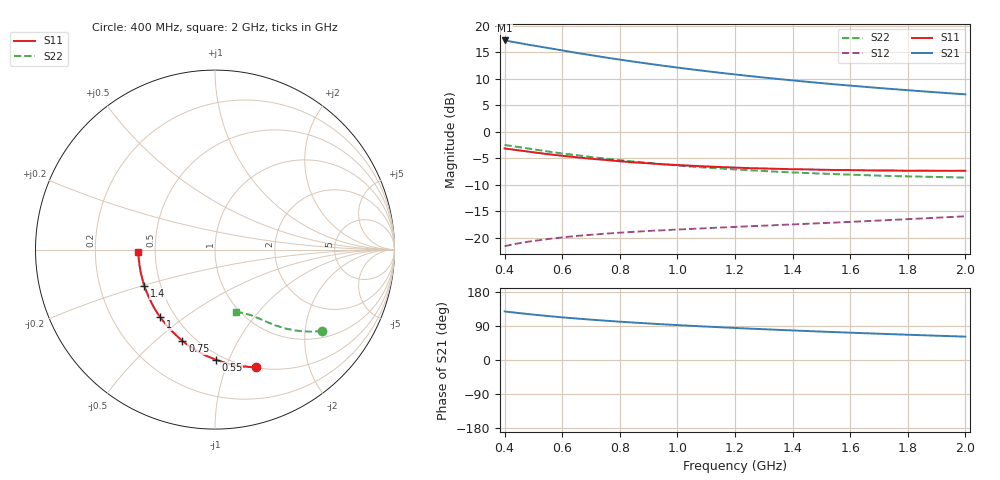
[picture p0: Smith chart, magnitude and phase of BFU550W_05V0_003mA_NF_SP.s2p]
! Filename:  P:\Prog\Test\Noise\ATS_data\Testdata_Net\06 Compressed Noise after Statistics\BFU550W_APM2013_11_D05_05p0V_003mA_NF_CM01_D.sf
! Date/Time: Tue 26/Mar/2013 16:25:22
! BFU550W_APM2013_11_D05_05p0V_1to35mA_NF_CM01_Bias3_R.sf
! Noise Parameter Data File
! BFU550W_APM2013_11_D05_05p0V_1to35mA_NF_CM01
! Date/time: Mon Mar 25 13:26:50 2013
! VAR V_out= 5.001000
! VAR I_out= 2.995000
! VAR V_in= 0.800700
! VAR I_in= 0.030605
! Device data file deembeded for feedlines and parallel
! Original file: \06 Compressed Noise after Statistics\BFU550W_APM2013_11_D05_05p0V_003mA_NF_CM01_R.sf
! Feed-files: PR019V01_070313_Feed1.s2p, PR019V01_070313_Feed2.s2p
! Parallel-file: PR019V01_070313_Par.s2p
# MHz S MA R 50
!  Freq-MHz  S11-mag  S11-arg  S21-mag  S21-arg  S12-mag  S12-arg  S22-mag  S22-arg
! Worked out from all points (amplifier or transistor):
!   37 points, 400 MHz to 2 GHz, reference 50 ohm
!   highest |S21| = 17.2 dB at 400 MHz (marker M1)
!   |S21| within 3 dB of that: start of sweep to 726.2 MHz
!   unconditionally stable (mu >= 1): 1.94 GHz to end of sweep
!   at 500 MHz: K = 0.37, MSG = 18.4 dB, |S12| = -20.6 dB
!   at 1.1 GHz: K = 0.73, MSG = 14.8 dB, |S12| = -18.2 dB
!   at 2 GHz: K = 1.01, MAG = 11.0 dB, |S12| = -16.0 dB
!   lowest NFmin = 0.48 dB at 420 MHz
!   S11 on the Smith chart (normalised r, x): 400 MHz: 0.51, -1.28; 550 MHz: 0.46, -0.90; 750 MHz: 0.43, -0.62; 1 GHz: 0.41, -0.41; 1.4 GHz: 0.41, -0.20; 2 GHz: 0.40, -0.01
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400  0.6947 -70.7  7.244 128.2  0.08316 54.9  0.7488 -37.0
440  0.671 -76.2  6.934 124.6  0.0876 53.0  0.7213 -39.2
480  0.6493 -81.2  6.622 121.4  0.09144 51.3  0.6945 -41.2
500  0.6385 -83.8  6.485 119.7  0.09316 50.6  0.6814 -42.0
550  0.6134 -89.6  6.157 116.0  0.09703 49.0  0.6504 -44.2
600  0.5922 -95.2  5.839 112.6  0.1006 47.6  0.6227 -45.9
650  0.5733 -100.1  5.53 109.5  0.1038 46.5  0.5997 -47.5
700  0.5552 -105.2  5.265 106.5  0.1065 45.5  0.5763 -49.1
750  0.5407 -109.6  5.006 103.8  0.1091 44.8  0.5564 -50.3
800  0.5253 -114.0  4.779 101.2  0.1114 44.3  0.5381 -51.6
850  0.513 -118.2  4.566 98.7  0.1136 43.8  0.5211 -52.6
900  0.5028 -122.0  4.37 96.4  0.1158 43.5  0.5072 -53.6
950  0.4922 -125.7  4.189 94.2  0.1175 43.3  0.4921 -54.6
1000  0.4843 -129.3  4.021 92.1  0.1194 43.2  0.4798 -55.4
1100  0.4698 -135.8  3.721 88.2  0.1229 43.2  0.4579 -57.2
1200  0.4582 -141.9  3.464 84.6  0.1264 43.5  0.4404 -58.9
1300  0.4494 -147.6  3.238 81.2  0.1298 43.9  0.4253 -60.4
1400  0.4423 -152.8  3.042 78.0  0.1333 44.5  0.4128 -61.8
1500  0.4372 -157.6  2.869 75.0  0.1371 45.2  0.4022 -63.4
1600  0.4338 -162.2  2.717 72.1  0.1409 46.0  0.393 -65.0
1750  0.4298 -168.4  2.518 68.0  0.1473 47.3  0.3811 -67.2
2000  0.4276 -178.1  2.248 61.6  0.1592 49.3  0.3689 -71.4
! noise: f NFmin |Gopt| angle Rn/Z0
400  0.5175  0.37  36.27  0.1277
460  0.4944  0.3626  40.72  0.1296
600  0.5621  0.357  50.29  0.131
800  0.6149  0.3375  67.36  0.1159
1000  0.6759  0.3471  81.81  0.1112
1200  0.7148  0.3497  95.89  0.1039
1400  0.7594  0.3842  114.3  0.0858
1600  0.7859  0.3593  125  0.0791
1800  0.8749  0.4249  141.9  0.0567
2000  0.8922  0.4455  154.2  0.0501
